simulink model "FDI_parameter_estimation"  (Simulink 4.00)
settings: Solver=FixedStepDiscrete  StartTime=0.0  StopTime=1000  RelTol=1e-3
libraries: slident x1, simulink3 x1

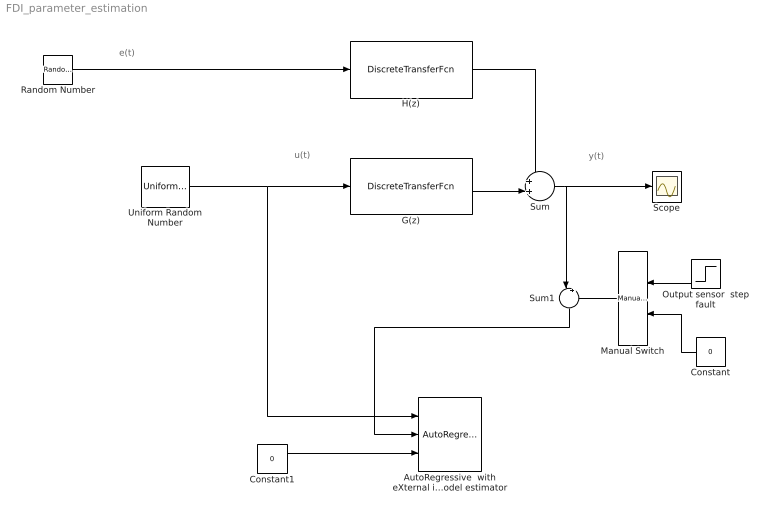
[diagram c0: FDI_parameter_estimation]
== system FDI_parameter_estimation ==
  note: y(t)
  note: e(t)
  note: u(t)
  AutoRegressive  with eXternal input model estimator : slident/AutoRegressive  with eXternal input model estimator
  Constant : Constant  Orientation=left  Value=0
  Constant1 : Constant  Value=0
  G(z) : DiscreteTransferFcn  Numerator=[0 1 0.5]  Denominator="[1  -1.5  0.7]"  SampleTime=1  Realization=auto
  H(z) : DiscreteTransferFcn  Numerator=[0 0 1]  Denominator="[1  -1.5  0.7]"  SampleTime=1  Realization=auto
  Manual Switch : simulink3/Nonlinear/Manual Switch  Orientation=left  sw=1  action=0
  Output sensor  step fault : Step  Orientation=left  Time=500  Before=0  After=1  SampleTime=1
  Random Number : RandomNumber  Mean=0  Variance=0.01  Seed=1  SampleTime=1
  Scope : Scope
  Sum : Sum  Inputs=++|  SaturateOnIntegerOverflow=on
  Sum1 : Sum  Orientation=down  Inputs=|++  SaturateOnIntegerOverflow=on
  Uniform Random Number : UniformRandomNumber  Minimum=-1  Maximum=1  Seed=0  SampleTime=1
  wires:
  G(z)/1 -> Sum/2
  H(z)/1 -> Sum/1
  Sum/1 -> Scope/1, Sum1/1
  Random Number/1 -> H(z)/1
  Sum1/1 -> AutoRegressive  with eXternal input model estimator/2
  Manual Switch/1 -> Sum1/2
  Output sensor  step fault/1 -> Manual Switch/1
  Constant/1 -> Manual Switch/2
  Uniform Random Number/1 -> AutoRegressive  with eXternal input model estimator/1, G(z)/1
  Constant1/1 -> AutoRegressive  with eXternal input model estimator/3
